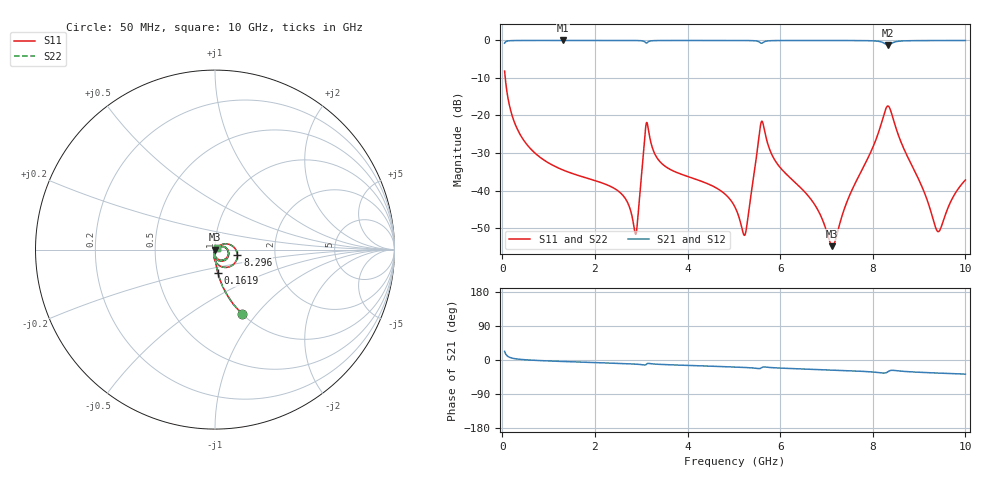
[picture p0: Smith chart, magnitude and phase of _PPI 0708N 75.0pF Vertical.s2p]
! S-Parameter data specifications (vertical orientation):
! Substrate: 40-mil Rogers 3003C, Substrate thickness, H=1.016mm, Dielectric constant, Er=3, Conductor thickness, T_mtl=0.043mm, Loss Tangent, Tand=0.003
! PCB Mounting Pad Footprint: Pad width, PadW=2.54mm , Pad length, PadL=0.51mm , Pad gap, PadG (edge-to-edge)=0.71mm , Reference planes=1.73mm apart
! Created Tue Jan 16 08:54:16 2018
# GHz S MA R 50
! 2 Port Network Data from SP1.SP block
! freq  magS11  angS11  magS21  angS21  magS12  angS12  magS22  angS22
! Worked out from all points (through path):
!   801 points, 50 MHz to 10 GHz, reference 50 ohm
!   highest |S21| = -0.01 dB at 1.306 GHz (marker M1); lowest = -1.2 dB at 8.333 GHz (marker M2)
!   group delay of S21, straight-line fit = 11 ps
!   lowest |S11| = -54.8 dB at 7.127 GHz (marker M3), VSWR 1.00, Z = 50.2 - j0.0949 ohm
!   |S11| at or under -10 dB: 63.6 MHz to end of sweep
!   |S22| runs from -54.8 to -8.2 dB; largest |S21 - S12| = 0
!   S11 on the Smith chart (normalised r, x): 50 MHz: 1.00, -0.85; 161.9 MHz: 1.00, -0.26; 8.296 GHz: 1.28, -0.08; 10 GHz: 1.02, +0.02
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0.05  0.3899 -67.2  0.9206 22.8  0.9206 22.8  0.3899 -67.2
0.1619375  0.13 -83.1  0.9913 6.8  0.9913 6.8  0.13 -83.1
0.5475  0.03986 -89.4  0.9989 0.2  0.9989 0.2  0.03986 -89.4
1.306188  0.01882 -92.6  0.9994 -3.9  0.9994 -3.9  0.01882 -92.6
1.716625  0.01534 -93.9  0.9993 -5.7  0.9993 -5.7  0.01534 -93.9
2.562375  0.009175 -94.0  0.999 -9.2  0.999 -9.2  0.009175 -94.0
2.873312  0.002625 -36.9  0.9975 -10.9  0.9975 -10.9  0.002625 -36.9
2.923062  0.00411 21.1  0.9964 -11.2  0.9964 -11.2  0.00411 21.1
3.109625  0.07911 -16.0  0.921 -11.5  0.921 -11.5  0.07911 -16.0
3.370812  0.02567 -95.1  0.9968 -11.3  0.9968 -11.3  0.02567 -95.1
4.664313  0.01043 -101.0  0.9987 -17.0  0.9987 -17.0  0.01043 -101.0
5.025  0.006003 -94.1  0.9983 -18.6  0.9983 -18.6  0.006003 -94.1
5.248875  0.002651 -15.6  0.9971 -19.8  0.9971 -19.8  0.002651 -15.6
5.609563  0.08393 -37.9  0.9197 -19.6  0.9197 -19.6  0.08393 -37.9
5.908062  0.02414 -101.8  0.9957 -20.8  0.9957 -20.8  0.02414 -101.8
6.691625  0.007259 -102.1  0.9981 -24.6  0.9981 -24.6  0.007259 -102.1
7.126938  0.001813 -31.5  0.9979 -26.5  0.9979 -26.5  0.001813 -31.5
8.296062  0.1283 -13.4  0.8779 -33.2  0.8779 -33.2  0.1283 -13.4
8.333375  0.1336 -33.0  0.8662 -30.4  0.8662 -30.4  0.1336 -33.0
8.345812  0.1317 -39.6  0.8698 -29.5  0.8698 -29.5  0.1317 -39.6
9.390562  0.002895 -41.7  0.9967 -34.4  0.9967 -34.4  0.002895 -41.7
10  0.01382 43.7  0.9973 -37.3  0.9973 -37.3  0.01382 43.7
